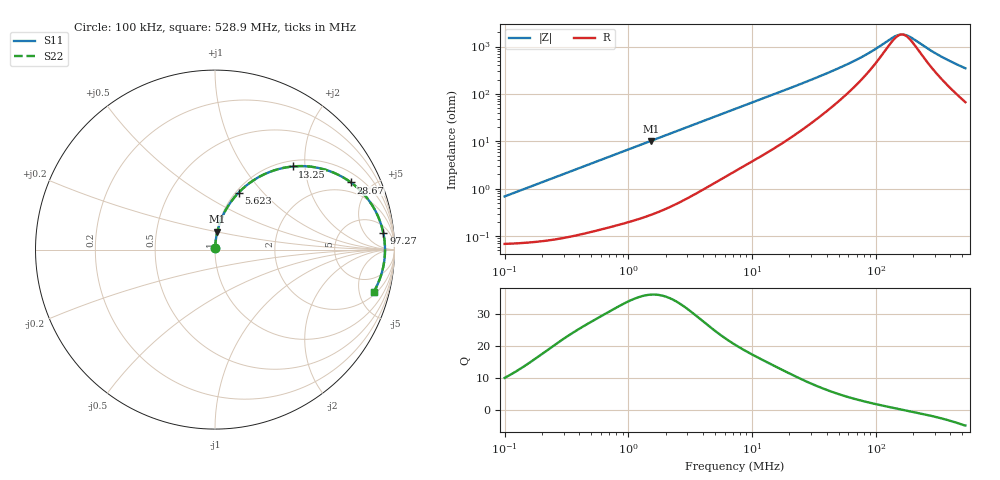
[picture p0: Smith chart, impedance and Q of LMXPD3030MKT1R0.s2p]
! LMXPD3030MKT1R0  S-PARAMETER MODEL  ( General Type )
! Model Generated by TAIYO YUDEN Corporation (http://www.ty-top.com)
! Version 1.0
! TAIYO YUDEN Control No. 191023NI43SB-FBB
! Copyright(c) 2019 TAIYO YUDEN CO.,LTD. All Rights Reserved.
! Product Description (link to TY-COMPAS)
! https://ds.yuden.co.jp/TYCOMPAS/or/detail?pn=LMXPD3030MKT1R0N&u=M
! Products Name : Inductors
! Characteristics :
!  Inductance : 1.0 uH , SRF(min) : 110 MHz , DC Resistance(max) : 0.078 Ohm
!  Rated Current : Saturation :2500 mA , Temp Rise : 1600 mA
!  Case Size : 3.0 x 3.0 / 0.118 x 0.118 [mm/inch] , Thickness : 1.2 / 0.047 [mm/inch]
!  (Conditions: Temperature = 25 degC , DC Bias Current/Voltage = 0A / 0V)
! External Node Assignments :
!  1  o---GGG---o  2
! GND o---------o GND
! Frequency Range : 0.1MHz  -  528.887669MHz  [ 402 STEP ]
# MHz S RI R 50
! Freq[MHz].  S11 Real  S11 Imag  S21 Real  S21 Imag  S12 Real  S12 Imag  S22 Real  S22 Imag
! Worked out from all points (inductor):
!   401 points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, 100 kHz to 528.9 MHz, reference 50 ohm
!   read as one part in series: L = 1.09 uH near 104.4 kHz
!   highest Q = 36.3 at 1.521 MHz (marker M1), where L = 1.06 uH
!   self-resonance near 162.3 MHz
!   S11 on the Smith chart (normalised r, x): 100 kHz: 1.00, +0.01; 5.623 MHz: 1.03, +0.74; 13.25 MHz: 1.12, +1.73; 28.67 MHz: 1.44, +3.76; 97.27 MHz: 9, +15; 528.9 MHz: 2.34, -6.81
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0.1  0.000731 0.00683  0.9993 -0.00683  0.9993 -0.00683  0.000731 0.00683
0.420401  0.00191 0.0284  0.9981 -0.0284  0.9981 -0.0284  0.00191 0.0284
1.521135  0.013 0.1001  0.987 -0.1001  0.987 -0.1001  0.013 0.1001
1.767367  0.0169 0.1157  0.9831 -0.1157  0.9831 -0.1157  0.0169 0.1157
3.434689  0.0559 0.2136  0.9441 -0.2136  0.9441 -0.2136  0.0559 0.2136
5.623165  0.1313 0.317  0.8687 -0.317  0.8687 -0.317  0.1313 0.317
7.430023  0.2039 0.379  0.7961 -0.379  0.7961 -0.379  0.2039 0.379
13.25309  0.4323 0.463  0.5677 -0.463  0.5677 -0.463  0.4323 0.463
19.0792  0.6001 0.4493  0.3999 -0.4493  0.3999 -0.4493  0.6001 0.4493
28.66948  0.7574 0.3741  0.2426 -0.3741  0.2426 -0.3741  0.7574 0.3741
30.5735  0.7772 0.3587  0.2228 -0.3587  0.2228 -0.3587  0.7772 0.3587
41.27269  0.8506 0.283  0.1494 -0.283  0.1494 -0.283  0.8506 0.283
58.15638  0.9022 0.1989  0.0978 -0.1989  0.0978 -0.1989  0.9022 0.1989
76.84342  0.9261 0.1377  0.0739 -0.1377  0.0739 -0.1377  0.9261 0.1377
97.27454  0.9381 0.091  0.0619 -0.091  0.0619 -0.091  0.9381 0.091
128.5312  0.9454 0.0404  0.0546 -0.0404  0.0546 -0.0404  0.9454 0.0404
152.5723  0.9471 0.0107  0.0529 -0.0107  0.0529 -0.0107  0.9471 0.0107
162.705  0.9472 -0.000412  0.0528 0.000412  0.0528 0.000412  0.9472 -0.000412
177.2697  0.947 -0.0152  0.053 0.0152  0.053 0.0152  0.947 -0.0152
197.3225  0.946 -0.0338  0.054 0.0338  0.054 0.0338  0.946 -0.0338
323.0502  0.9303 -0.1257  0.0697 0.1257  0.0697 0.1257  0.9303 -0.1257
528.8877  0.8838 -0.2369  0.1162 0.2369  0.1162 0.2369  0.8838 -0.2369
